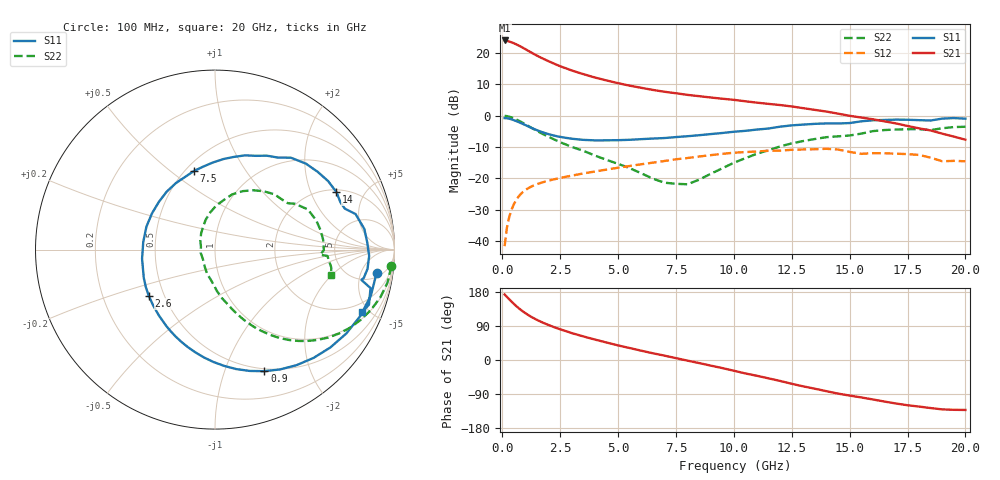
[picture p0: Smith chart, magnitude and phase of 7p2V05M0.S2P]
! Infineon Technologies  Discrete & RF Semiconductors
! bfp620
! VCE =  2.0 V,  IC =  5.0 mA
! Common Emitter S-Parameters:  Sep 2002
# GHz  S  MA  R  50
!  f  S11  S21  S12  S22
! GHz  MAG  ANG  MAG  ANG  MAG  ANG  MAG  ANG
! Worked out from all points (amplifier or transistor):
!   59 points, 100 MHz to 20 GHz, reference 50 ohm
!   highest |S21| = 23.9 dB at 100 MHz (marker M1)
!   |S21| within 3 dB of that: start of sweep to 1.052 GHz
!   unconditionally stable (mu >= 1): 4.809 GHz to 11.69 GHz; 14.69 GHz to 15.31 GHz; 17.18 GHz to end of sweep
!   at 1 GHz: K = 0.32, MSG = 22.4 dB, |S12| = -23.7 dB
!   at 5.5 GHz: K = 1.04, MAG = 11.5 dB, |S12| = -16.1 dB
!   at 20 GHz: K = 1.34, MAG = -0.1 dB, |S12| = -14.6 dB
!   S11 on the Smith chart (normalised r, x): 100 MHz: 6, -10; 900 MHz: 0.47, -1.38; 2.6 GHz: 0.41, -0.27; 7.5 GHz: 0.55, +0.61; 14 GHz: 2.13, +3.09; 20 GHz: 1.35, -4.56
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0.1  0.9096 -8.2  15.69 172.9  0.0083 79.2  0.9868 -5.4
0.2  0.9056 -16.5  15.46 166.5  0.0163 79.5  0.9785 -10.8
0.3  0.89 -24.6  15.09 160.2  0.0242 76.2  0.9592 -16.0
0.4  0.8681 -32.6  14.64 154.0  0.0317 72.3  0.9327 -21.0
0.5  0.8429 -40.3  14.15 148.1  0.0387 68.5  0.9017 -25.7
0.7  0.788 -54.8  13.07 137.2  0.051 61.6  0.8323 -34.3
0.9  0.7312 -67.9  11.95 127.8  0.0609 55.6  0.7597 -41.5
1.1  0.6762 -79.9  10.85 119.5  0.0688 50.6  0.6891 -47.6
1.3  0.6262 -90.8  9.851 112.2  0.0753 46.5  0.6245 -52.7
1.6  0.5646 -105.4  8.603 102.8  0.0831 41.9  0.5425 -58.7
2  0.5051 -122.4  7.328 92.3  0.0917 37.5  0.458 -65.0
2.6  0.45 -145.0  5.901 79.0  0.1031 32.6  0.363 -72.4
3  0.427 -158.3  5.216 71.0  0.1103 29.9  0.3162 -76.5
3.5  0.4095 -172.9  4.563 62.2  0.1196 26.9  0.2743 -81.7
5  0.405 150.0  3.276 38.5  0.1474 18.0  0.1701 -97.8
7  0.4379 112.3  2.393 11.6  0.1886 4.8  0.0852 -143.1
7.5  0.4536 105.0  2.263 4.9  0.2008 0.7  0.0817 -167.0
10.5  0.5705 66.3  1.686 -35.5  0.2619 -28.0  0.2095 97.1
13.5  0.7369 31.2  1.23 -75.8  0.2905 -58.7  0.4227 50.3
14  0.7487 25.3  1.156 -82.3  0.295 -65.0  0.4522 43.0
17  0.8597 -2.4  0.749 -114.8  0.2467 -89.4  0.5983 10.3
20  0.8916 -22.9  0.412 -131.8  0.1868 -103.5  0.6625 -12.3
